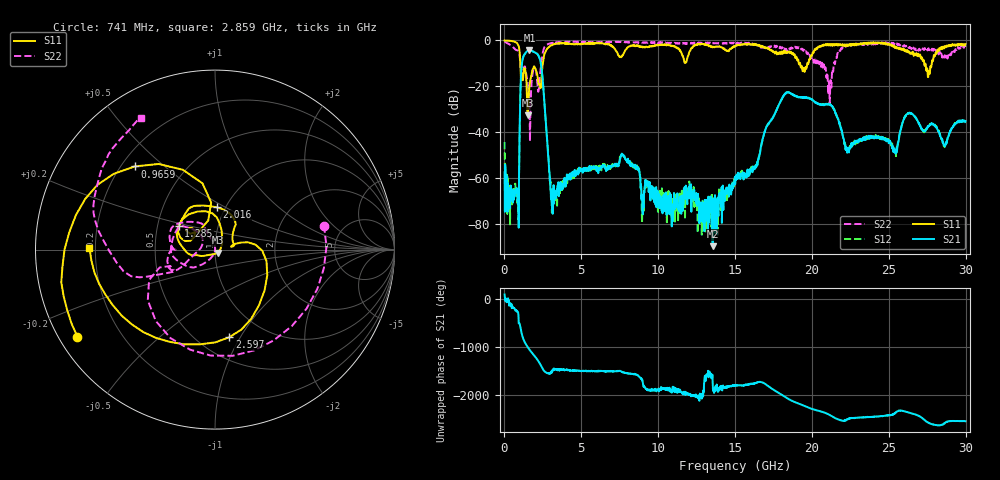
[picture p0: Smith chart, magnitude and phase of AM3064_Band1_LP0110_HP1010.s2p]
# Hz S DB R 50.0
!freq dBS11 angS11 dBS21 angS21 dBS12 angS12 dBS22 angS22
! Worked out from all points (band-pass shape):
!   1600 points, 10 MHz to 29.98 GHz, reference 50 ohm
!   highest |S21| = -4.36 dB at 1.622 GHz (marker M1); lowest = -89.8 dB at 13.54 GHz (marker M2)
!   |S21| within 3 dB of the highest: 1.217 GHz to 2.263 GHz (1.046 GHz wide, 60.1 % of centre)
!   lowest |S11| = -32.7 dB at 1.51 GHz (marker M3), VSWR 1.05, Z = 51.5 - j1.8 ohm
!   |S11| at or under -10 dB: 1.031 GHz to 2.498 GHz (1.467 GHz wide, 83.1 % of centre); 19.23 GHz to 19.7 GHz (473.2 MHz wide, 2.43 % of centre); 27.3 GHz to 27.79 GHz (491.8 MHz wide, 1.79 % of centre)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
!   |S22| runs from -44.0 to -0.4 dB; largest |S21 - S12| = 0.007
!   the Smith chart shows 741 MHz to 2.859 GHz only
!   S11 on the Smith chart (normalised r, x): 741 MHz: 0.05, -0.29; 965.9 MHz: 0.25, +0.40; 1.285 GHz: 0.64, +0.18; 2.016 GHz: 0.91, +0.45; 2.597 GHz: 0.70, -0.90; 2.859 GHz: 0.18, +0.01
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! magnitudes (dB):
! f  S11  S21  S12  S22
! 10 MHz  0.0  -57.6  -44.4  -0.4
! 741 MHz  -0.8  -66.4  -66.8  -4.1
! 965.9 MHz  -3.8  -48.5  -48.2  -5.7
! 1.285 GHz  -12.3  -6.3  -6.3  -11.6
! 1.51 GHz  -32.7  -4.5  -4.5  -18.5
! 1.622 GHz  -20.3  -4.4  -4.3  -27.8
! 2.016 GHz  -12.5  -5.4  -5.3  -12.5
! 2.597 GHz  -6.1  -27.0  -27.0  -3.0
! 2.859 GHz  -3.1  -50.9  -51.1  -1.5
! 3.196 GHz  -1.6  -63.2  -70.7  -1.1
! 5.015 GHz  -1.6  -56.2  -56.2  -0.7
! 7.714 GHz  -6.3  -50.2  -49.9  -0.7
! 10 GHz  -2.1  -66.4  -67.7  -0.9
! 13.54 GHz  -3.0  -89.8  -70.5  -1.2
! 15 GHz  -2.6  -62.8  -60.4  -1.5
! 18.25 GHz  -5.0  -23.3  -23.2  -4.3
! 19.99 GHz  -6.7  -25.8  -25.8  -8.2
! 21.15 GHz  -1.8  -28.0  -27.8  -27.5
! 22.3 GHz  -2.4  -49.0  -48.3  -2.3
! 25 GHz  -1.5  -44.9  -44.3  -1.2
! 27.56 GHz  -16.0  -37.4  -37.3  -3.6
! 29.98 GHz  -1.6  -35.3  -35.1  -2.8
